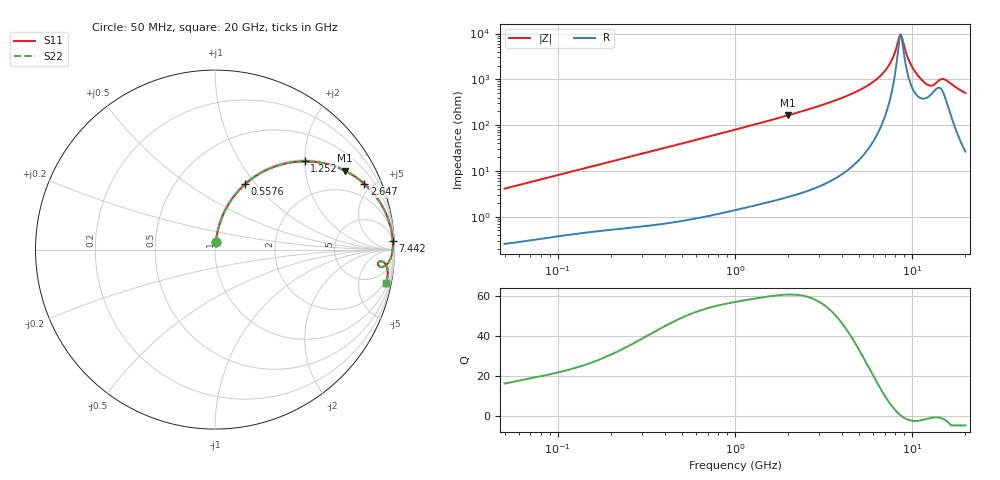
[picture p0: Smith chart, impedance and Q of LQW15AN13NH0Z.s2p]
!Murata Part Number: LQW15AN13NH0Z
!These Parameters are Measured in Series Mode Connection
!  o--[Z]--o
!Port1  Port2
!  o-------o
!Freq. Start=50[MHz] Stop=20[GHz], 401[Steps]
# Hz S RI R 50
!Freq.(Hz) S11(Real) S11(Imag) S21(Real) S21(Imag) S12(Real) S12(Imag) S22(Real) S22(Imag)
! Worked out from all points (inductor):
!   401 points, 50 MHz to 20 GHz, reference 50 ohm
!   read as one part in series: L = 13 nH near 51.52 MHz
!   highest Q = 60.9 at 1.992 GHz (marker M1), where L = 13 nH
!   self-resonance near 8.516 GHz
!   S11 on the Smith chart (normalised r, x): 50 MHz: 1.01, +0.08; 557.6 MHz: 1.02, +0.88; 1.252 GHz: 1.03, +2.00; 2.647 GHz: 1.08, +4.52; 7.442 GHz: 7, +41; 20 GHz: 2, -10
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5e7  0.00419 0.0406  0.9958 -0.0406  0.9958 -0.0406  0.00419 0.0406
1.364002e8  0.016 0.107  0.984 -0.107  0.984 -0.107  0.016 0.107
3.721004e8  0.0849 0.2675  0.9151 -0.2675  0.9151 -0.2675  0.0849 0.2675
5.575697e8  0.1674 0.3636  0.8326 -0.3636  0.8326 -0.3636  0.1674 0.3636
1e9  0.3882 0.4787  0.6118 -0.4787  0.6118 -0.4787  0.3882 0.4787
1.251922e9  0.4992 0.4916  0.5008 -0.4916  0.5008 -0.4916  0.4992 0.4916
1.99176e9  0.724 0.4389  0.276 -0.4389  0.276 -0.4389  0.724 0.4389
2.647493e9  0.8319 0.3656  0.1681 -0.3656  0.1681 -0.3656  0.8319 0.3656
2.728004e9  0.8414 0.3569  0.1586 -0.3569  0.1586 -0.3569  0.8414 0.3569
4.026975e9  0.9349 0.2362  0.0651 -0.2362  0.0651 -0.2362  0.9349 0.2362
5.352748e9  0.9724 0.1473  0.0276 -0.1473  0.0276 -0.1473  0.9724 0.1473
6.503449e9  0.9862 0.0877  0.0138 -0.0877  0.0138 -0.0877  0.9862 0.0877
7.442007e9  0.9906 0.0465  0.00942 -0.0465  0.00942 -0.0465  0.9906 0.0465
7.901521e9  0.991 0.0279  0.00897 -0.0279  0.00897 -0.0279  0.991 0.0279
8.389408e9  0.9904 0.00911  0.00959 -0.00911  0.00959 -0.00911  0.9904 0.00911
8.644534e9  0.9896 -0.000404  0.0104 0.000404  0.0104 0.000404  0.9896 -0.000404
8.774992e9  0.9891 -0.00519  0.0109 0.00519  0.0109 0.00519  0.9891 -0.00519
9.892087e9  0.9805 -0.0444  0.0195 0.0444  0.0195 0.0444  0.9805 -0.0444
1.149051e10  0.9487 -0.0899  0.0513 0.0899  0.0513 0.0899  0.9487 -0.0899
1.276073e10  0.9109 -0.0892  0.0891 0.0892  0.0891 0.0892  0.9109 -0.0892
1.504638e10  0.9474 -0.0779  0.0526 0.0779  0.0526 0.0779  0.9474 -0.0779
2e10  0.9526 -0.1877  0.0474 0.1877  0.0474 0.1877  0.9526 -0.1877
